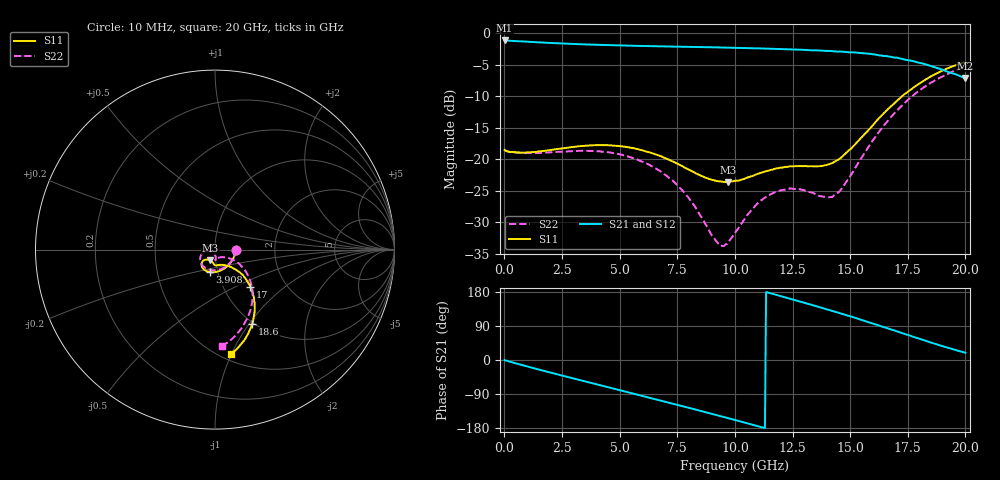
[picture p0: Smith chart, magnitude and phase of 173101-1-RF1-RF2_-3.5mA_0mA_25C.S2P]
!  2-Port S-parameters saved by WinCal
! VAR NAME=173101-1-RF1-RF2_-3.5mA_0mA_25C
! VAR DATE=2017-7-20 9:33:51
! VAR FILENAME=173101-1-RF1-RF2_-3.5mA_0mA_25C.S2P
! VAR MeasName=S-Parameters (CALIBRATED_DATA) read from VNA (N5242A)
! VAR MeasDate=2017-7-20 9:32:27
! VAR PHYS_PORTS=1,2
# Hz S DB R 50
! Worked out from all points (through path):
!   401 points, 10 MHz to 20 GHz, reference 50 ohm
!   highest |S21| = -1.18 dB at 10 MHz (marker M1); lowest = -7.1 dB at 20 GHz (marker M2)
!   group delay of S21, straight-line fit = 46.8 ps
!   lowest |S11| = -23.6 dB at 9.705 GHz (marker M3), VSWR 1.14, Z = 47 - j5.66 ohm
!   |S11| at or under -10 dB: start of sweep to 17.26 GHz
!   |S22| runs from -33.8 to -5.4 dB; largest |S21 - S12| = 0.0067
!   S11 on the Smith chart (normalised r, x): 10 MHz: 1.27, -0.00; 3.908 GHz: 0.91, -0.23; 17 GHz: 1.34, -0.60; 18.6 GHz: 0.98, -1.04; 20 GHz: 0.56, -1.00
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1e7  -18.55 -0.9  -1.18 -0.2  -1.18 -0.2  -18.52 -0.9
1.50925e9  -18.77 -53.2  -1.48 -25.5  -1.49 -25.5  -19.03 -55.6
3.358325e9  -17.92 -94.7  -1.79 -54.3  -1.79 -54.2  -18.67 -103.1
3.90805e9  -17.79 -103.7  -1.85 -62.7  -1.86 -62.7  -18.71 -114.3
5.357325e9  -18.11 -123.0  -2.00 -85.0  -2.02 -84.9  -19.58 -140.1
6.70665e9  -19.44 -134.6  -2.11 -105.9  -2.10 -105.7  -21.77 -159.5
7.856075e9  -21.40 -136.4  -2.19 -123.8  -2.20 -123.7  -25.51 -169.5
9.255375e9  -23.50 -122.0  -2.28 -146.2  -2.28 -146.1  -33.28 -140.6
9.70515e9  -23.65 -114.2  -2.32 -153.5  -2.32 -153.4  -33.21 -111.4
1.0005e10  -23.44 -109.3  -2.36 -158.4  -2.36 -158.3  -31.67 -97.1
1.085458e10  -22.52 -98.3  -2.43 -172.3  -2.44 -172.2  -27.53 -84.3
1.155422e10  -21.71 -94.0  -2.50 176.0  -2.50 176.1  -25.57 -85.6
1.235382e10  -21.16 -90.3  -2.59 162.4  -2.60 162.6  -24.67 -87.8
1.335332e10  -21.13 -81.9  -2.74 145.1  -2.72 145.4  -25.32 -84.3
1.410295e10  -20.80 -67.9  -2.84 131.7  -2.86 131.8  -26.04 -66.2
1.450275e10  -20.02 -59.2  -2.95 124.6  -2.95 124.7  -25.18 -50.8
1.570215e10  -15.75 -43.7  -3.24 101.7  -3.27 102.0  -18.58 -29.2
1.670165e10  -11.88 -44.7  -3.73 82.0  -3.77 82.0  -13.64 -35.1
1.70015e10  -10.85 -46.4  -3.89 76.2  -3.89 76.4  -12.39 -38.8
1.78011e10  -8.51 -54.0  -4.52 60.0  -4.52 60.2  -9.70 -50.3
1.86007e10  -6.69 -63.3  -5.35 44.2  -5.38 44.5  -7.68 -63.2
2e10  -4.59 -81.4  -7.14 19.0  -7.19 19.7  -5.35 -85.9
